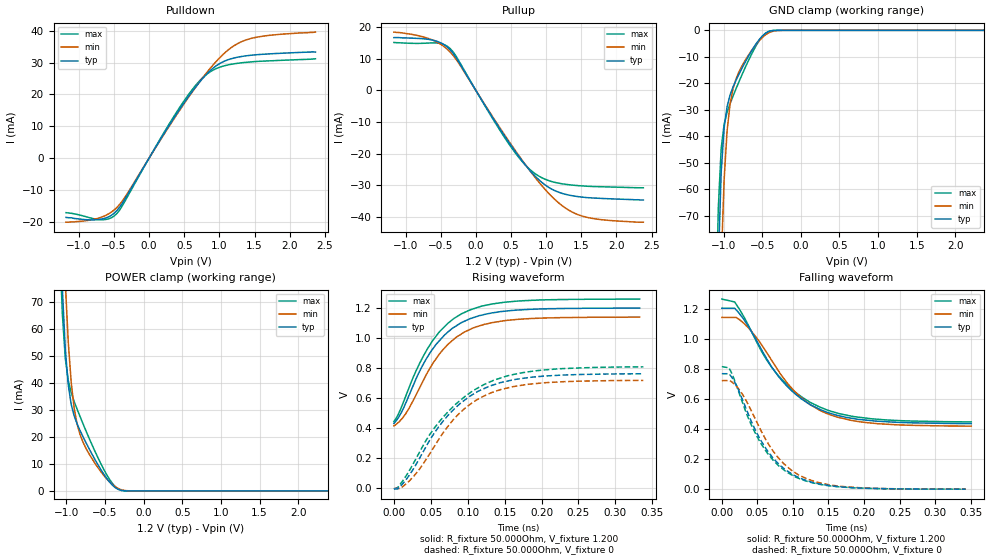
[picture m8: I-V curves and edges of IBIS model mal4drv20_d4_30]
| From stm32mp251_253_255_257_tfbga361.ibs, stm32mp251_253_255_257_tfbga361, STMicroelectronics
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[Model] mal4drv20_d4_30
Model_type   I/O
Polarity   Non-Inverting
Enable   Active-High
C_comp   1.838pF   1.835pF   1.848pF
C_comp_pullup   938.881fF   931.604fF   947.115fF
C_comp_pulldown 782.410fF   779.859fF   796.520fF
Vinh = 668.000mV
Vinl = 532.000mV
Vmeas = 600.000mV
Vref = 600.000mV
Rref = 50Ohms
Cref = 0pF
[Model Spec]
Vinh   668.000mV   638.000mV   698.000mV
Vinl   532.000mV   502.000mV   562.000mV
Vmeas   600.000mV   570.000mV   630.000mV
Vref   600.000mV   570.000mV   630.000mV
D_overshoot_ampl_h 0.24 NA   NA
D_overshoot_ampl_l 0.24 NA   NA
D_overshoot_area_l 300.000m NA   NA
D_overshoot_area_h 300.000m NA   NA
[Receiver Thresholds]
Vth = 600.000mV
Vth_min = 570.000mV
Vth_max = 630.000mV
Vinh_ac = 68.000mV
Vinh_dc = 68.000mV
Vinl_ac = -68.000mV
Vinl_dc = -68.000mV
Tslew_ac = 5.000ns
Threshold_sensitivity = 0.5
Reference_supply Pullup_ref
[Temperature Range]   25.000   125.000   -40.000
[Voltage Range]   1.200V   1.140V   1.260V
[GND Clamp Reference]   0.00V   0.00V   0.00V
[C Comp Corner]
| variable   typ   min   max
C_comp 1.848pF   1.838pF   1.835pF
C_comp_pullup 938.881fF   947.115fF   931.604fF
C_comp_pulldown 779.859fF   796.520fF   782.410fF
[Pulldown Reference]   0.00V   0.00V   0.00V
[POWER Clamp Reference]   1.200V   1.140V   1.260V
[Pullup Reference]   1.200V   1.140V   1.260V
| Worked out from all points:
|   slope of the pulldown table from 0 to 0.18 V, typ, clamps not added: 27.5 ohm
|   slope of the pullup table from 0 to 0.18 V, typ, clamps not added: 27.8 ohm
|   GND clamp passes 1 mA (typ) near -0.45 V on its own axis
|   POWER clamp passes 1 mA (typ) near -0.35 V on its own axis
|   rising waveform, R_fixture 50.000Ohm, V_fixture 1.200: 20-80 % time 57ps typ, 58.2ps min, 57.3ps max; typ from 0.433 V to 1.2 V
|   rising waveform, R_fixture 50.000Ohm, V_fixture 0: 20-80 % time 72.8ps typ, 70.7ps min, 80.5ps max; typ from -0.003 V to 0.763 V
|   falling waveform, R_fixture 50.000Ohm, V_fixture 1.200: 20-80 % time 73.9ps typ, 73.3ps min, 77ps max; typ from 1.2 V to 0.436 V
|   falling waveform, R_fixture 50.000Ohm, V_fixture 0: 20-80 % time 55.7ps typ, 57.7ps min, 55.1ps max; typ from 0.767 V to 0 V
[GND Clamp]
-1.184V   -365mA     -429.3mA   -336.5mA
-1.107V   -152.4mA   -215.7mA   -121.1mA
-1.069V   -88.87mA   -140.5mA   -67.62mA
-1.031V   -53.54mA   -88.39mA   -44.48mA
-992.7mV  -36.7mA    -56.18mA   -35.42mA
-954.6mV  -28.78mA   -37.93mA   -30.92mA
-916.4mV  -24.43mA   -27.89mA   -27.7mA
-840mV    -18.89mA   -18.42mA   -22.12mA
-763.6mV  -14.38mA   -13.51mA   -16.88mA
-572.7mV  -4.818mA   -5.067mA   -5.477mA
-458.2mV  -1.146mA   -1.695mA   -1.103mA
2.367V    25.44nA    625nA      8.401nA
[Power Clamp]
-1.167V   197.6mA    234.2mA    183.1mA
-1.091V   108mA      144mA      94.42mA
-1.053V   75.21mA    107.2mA    65.93mA
-1.015V   52.65mA    77.42mA    49.33mA
-976.4mV  39.37mA    55.31mA    41.02mA
-938.2mV  32.15mA    40.29mA    36.48mA
-900mV    27.91mA    30.75mA    33.22mA
-823.6mV  22.42mA    20.91mA    27.62mA
-632.7mV  11.76mA    10.36mA    14.83mA
-365.4mV  1.178mA    1.496mA    1.508mA
-212.7mV  14.35uA    76.22uA    9.056uA
2.384V    -16.74nA   -562.7nA   -5.86nA
[Pulldown]
-1.184V   -18.7mA    -20.2mA    -17.2mA
-725.5mV  -19.38mA   -18.95mA   -19.34mA
-572.7mV  -18.46mA   -17.51mA   -19.11mA
-458.2mV  -16.51mA   -15.53mA   -17.43mA
-343.6mV  -12.87mA   -12.29mA   -13.55mA
152.7mV   5.565mA    5.403mA    5.829mA
496.4mV   17.32mA    17.05mA    17.94mA
725.5mV   24.09mA    24.17mA    24.44mA
954.5mV   29mA       30.37mA    28.12mA
1.184V    31.31mA    34.95mA    29.53mA
1.413V    32.23mA    37.37mA    30.15mA
2.367V    33.3mA     39.6mA     31.2mA
[Pullup]
-1.167V   16.7mA     18.44mA    15.16mA
-594.5mV  15.8mA     15.71mA    15.03mA
-480mV    14.82mA    14.3mA     14.7mA
-365.4mV  12.83mA    12.13mA    13.22mA
-289.1mV  10.61mA    10.06mA    11.07mA
474.6mV   -16.54mA   -16.19mA   -17.03mA
703.6mV   -23.51mA   -23.4mA    -23.54mA
894.5mV   -28.17mA   -28.89mA   -27.02mA
1.2V      -32.3mA    -35.9mA    -29.37mA
1.467V    -33.56mA   -39.34mA   -30.07mA
1.773V    -34.07mA   -40.77mA   -30.4mA
2.384V    -34.6mA    -41.6mA    -30.74mA
[Ramp]
R_load=50.000Ohm
dV/dt_r   458.820mV/66.000ps  432.779mV/65.500ps  487.410mV/70.000ps
dV/dt_f   458.820mV/66.000ps  432.779mV/67.000ps  487.410mV/67.000ps
[Rising waveform]
R_fixture=50.000Ohm
V_fixture=1.200
V_fixture_min=1.140
V_fixture_max=1.260
0s        432.7mV    416.4mV    444.7mV
9ps       494.5mV    453mV      526.5mV
19ps      602.1mV    520.5mV    653.1mV
33ps      761.1mV    652.5mV    814.1mV
49ps      902.5mV    801.7mV    956.7mV
72ps      1.036V     952.7mV    1.093V
92ps      1.104V     1.03V      1.163V
122ps     1.157V     1.091V     1.216V
158ps     1.183V     1.121V     1.242V
333ps     1.2V       1.14V      1.26V
[Rising waveform]
R_fixture=50.000Ohm
V_fixture=0
0s        -3.289mV   -842.7uV   -5.177mV
9ps       15.11mV    2.217mV    30.31mV
25ps      118.4mV    70.44mV    153.2mV
47ps      308.3mV    218.8mV    346.9mV
66ps      444.2mV    365.5mV    470.6mV
94ps      580.8mV    524.1mV    603.7mV
120ps     659.6mV    610mV      686.5mV
160ps     721.1mV    676.2mV    756.4mV
198ps     745.1mV    701.1mV    786.1mV
338ps     762.8mV    718.8mV    809mV
[Falling waveform]
R_fixture=50.000Ohm
V_fixture=1.200
V_fixture_min=1.140
V_fixture_max=1.260
0s        1.202V     1.141V     1.263V
18ps      1.202V     1.141V     1.244V
33ps      1.114V     1.093V     1.128V
55ps      934mV      965.6mV    923mV
76ps      772mV      811.2mV    774.3mV
107ps     618.2mV    627.5mV    631.4mV
136ps     533.4mV    528.4mV    549mV
162ps     490.9mV    479.1mV    506.3mV
199ps     460.4mV    444.6mV    473.8mV
351ps     435.7mV    418.9mV    447.2mV
[Falling waveform]
R_fixture=50.000Ohm
V_fixture=0
0s        767.1mV    721.5mV    814.2mV
10ps      767.1mV    721.5mV    806.5mV
17ps      721.2mV    700.4mV    734.4mV
36ps      511.2mV    572.6mV    486.7mV
56ps      315mV      380.6mV    296.4mV
78ps      176.9mV    216.7mV    164.8mV
101ps     93.73mV    116.3mV    86.93mV
133ps     39.19mV    47.41mV    36.64mV
173ps     13.49mV    16.24mV    12.79mV
343ps     219.1uV    325.6uV    190.9uV
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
